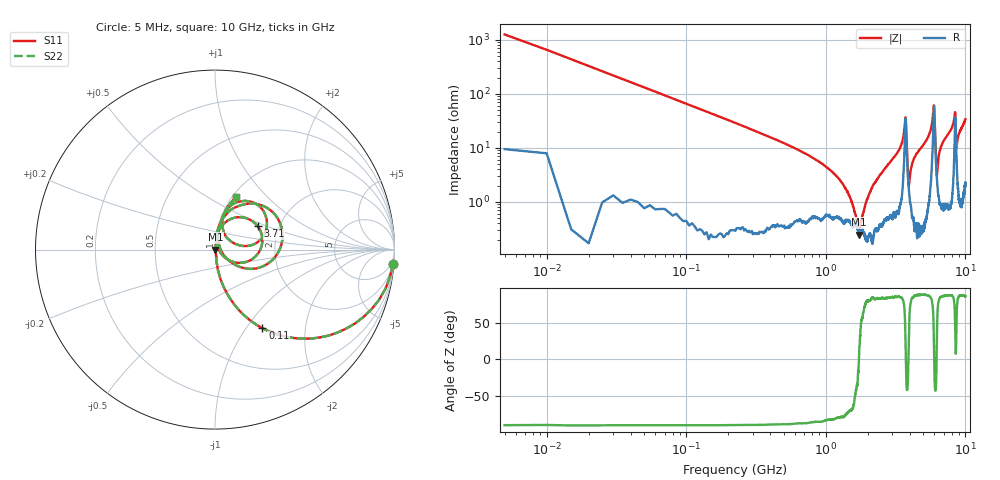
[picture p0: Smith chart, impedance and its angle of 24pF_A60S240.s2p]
! Amotech Co.,Ltd.
! http://www.amotech.co.kr/
! Part Number: A60S240
! These Parameters are Measured in Series Mode Connection
! Operation Temp=25[degC], DC Bias Voltage=0[V]
! Freq. Start=5[MHz] Stop=10[GHz], 2000[Steps]
! Date: Monday, July 13, 2020, 01:39:12
# GHZ S RI R 50.000000
!Freq.(Hz) S11(Real) S11(Imag) S21(Real) S21(Imag) S12(Real) S12(Imag) S22(Real) S22(Imag)
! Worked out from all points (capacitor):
!   2000 points, 5 MHz to 10 GHz, reference 50 ohm
!   read as one part in series: C = 24.2 pF near 55 MHz
!   lowest |Z| = 250 mohm at 1.735 GHz (marker M1)
!   series resonance near 1.728 GHz, so ESL is about 350 pH
!   S11 on the Smith chart (normalised r, x): 5 MHz: 1, -25; 110 MHz: 1.01, -1.19; 3.71 GHz: 1.55, +0.44; 10 GHz: 1.05, +0.67
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0.005  0.9931 -0.0793  0.00693 0.0793  0.00693 0.0793  0.9931 -0.0793
0.065  0.5056 -0.4963  0.4944 0.4963  0.4944 0.4963  0.5056 -0.4963
0.11  0.2638 -0.4373  0.7362 0.4373  0.7362 0.4373  0.2638 -0.4373
0.325  0.0399 -0.1891  0.9601 0.1891  0.9601 0.1891  0.0399 -0.1891
1.335  0.00447 -0.0202  0.9955 0.0202  0.9955 0.0202  0.00447 -0.0202
1.675  0.00368 -0.00239  0.9963 0.00239  0.9963 0.00239  0.00368 -0.00239
1.735  0.00244 0.000514  0.9976 -0.000514  0.9976 -0.000514  0.00244 0.000514
2.175  0.00225 0.0201  0.9977 -0.0201  0.9977 -0.0201  0.00225 0.0201
3.34  0.0149 0.0886  0.9851 -0.0886  0.9851 -0.0886  0.0149 0.0886
3.71  0.2376 0.1307  0.7624 -0.1307  0.7624 -0.1307  0.2376 0.1307
3.935  0.017 0.0103  0.983 -0.0103  0.983 -0.0103  0.017 0.0103
4.26  0.00847 0.0608  0.9915 -0.0608  0.9915 -0.0608  0.00847 0.0608
5.005  0.0158 0.1129  0.9842 -0.1129  0.9842 -0.1129  0.0158 0.1129
5.695  0.0756 0.2117  0.9244 -0.2117  0.9244 -0.2117  0.0756 0.2117
5.93  0.3554 0.1631  0.6446 -0.1631  0.6446 -0.1631  0.3554 0.1631
6.035  0.2065 -0.1075  0.7935 0.1075  0.7935 0.1075  0.2065 -0.1075
6.235  0.0287 0.00836  0.9713 -0.00836  0.9713 -0.00836  0.0287 0.00836
6.67  0.0189 0.1003  0.9811 -0.1003  0.9811 -0.1003  0.0189 0.1003
8.335  0.1659 0.2715  0.8341 -0.2715  0.8341 -0.2715  0.1659 0.2715
8.455  0.2894 0.1482  0.7106 -0.1482  0.7106 -0.1482  0.2894 0.1482
8.64  0.0635 0.07  0.9365 -0.07  0.9365 -0.07  0.0635 0.07
10  0.1183 0.2908  0.8817 -0.2908  0.8817 -0.2908  0.1183 0.2908
